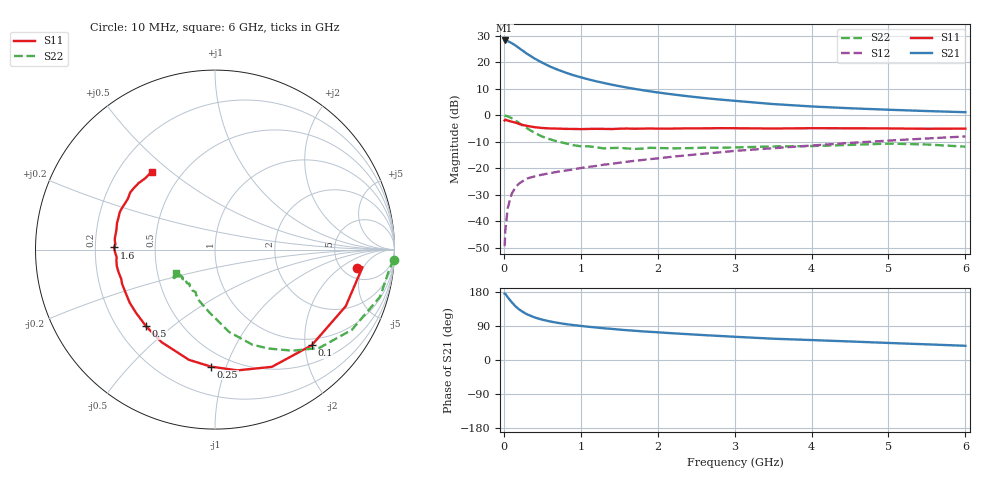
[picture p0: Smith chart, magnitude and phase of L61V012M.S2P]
!  INFINEON TECHNOLOGIES Small Signal Semiconductors
! BFR380L3 , Si-NPN RF-Transistor in TSLP-3-1
!  Vce=1 V,  Ic=12.5 mA
! Common Emitter S-Parameters:  07. March 2005
#  GHz  S  MA  R  50
! f  S11  S21  S12  S22
! GHz  Mag  Ang  Mag  Ang  Mag  Ang  Mag  Ang
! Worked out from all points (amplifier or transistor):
!   36 points, 10 MHz to 6 GHz, reference 50 ohm
!   highest |S21| = 28.2 dB at 10 MHz (marker M1)
!   |S21| within 3 dB of that: start of sweep to 204.1 MHz
!   unconditionally stable (mu >= 1): 1.958 GHz to 4.989 GHz
!   at 250 MHz: K = 0.30, MSG = 24.5 dB, |S12| = -24.7 dB
!   at 1.4 GHz: K = 0.92, MSG = 14.9 dB, |S12| = -18.3 dB
!   at 6 GHz: K = 0.98, MSG = 4.6 dB, |S12| = -8.0 dB
!   S11 on the Smith chart (normalised r, x): 10 MHz: 6.80, -3.73; 100 MHz: 0.86, -2.15; 250 MHz: 0.39, -0.89; 500 MHz: 0.32, -0.41; 1.6 GHz: 0.28, +0.01; 6 GHz: 0.34, +0.43
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0.01  0.7976 -7.2  25.7 175.3  0.0034 86.0  0.9993 -3.2
0.02  0.8273 -6.8  25.59 174.4  0.0069 90.8  0.9769 -6.6
0.05  0.7938 -23.4  24.94 165.7  0.0176 80.1  0.9566 -15.9
0.1  0.7579 -44.7  22.99 153.0  0.0325 69.3  0.8838 -30.4
0.15  0.7261 -64.1  20.74 141.9  0.0438 61.5  0.7985 -43.3
0.2  0.6845 -79.4  18.37 133.2  0.0519 56.3  0.7109 -52.4
0.25  0.6524 -92.0  16.31 126.5  0.058 51.5  0.6273 -61.5
0.3  0.6311 -103.3  14.46 120.7  0.064 49.3  0.5696 -68.5
0.4  0.5954 -120.0  11.72 112.3  0.0704 46.2  0.4644 -80.4
0.5  0.5744 -132.0  9.767 106.4  0.076 45.7  0.396 -87.8
0.6  0.5638 -141.3  8.278 101.7  0.081 45.7  0.3521 -95.0
0.7  0.5599 -148.0  7.225 98.1  0.086 46.6  0.3187 -101.7
0.9  0.5518 -159.8  5.707 92.3  0.095 48.4  0.2731 -112.6
1.1  0.5518 -166.8  4.743 87.7  0.1062 50.7  0.26 -119.1
1.4  0.5495 -175.6  3.774 82.2  0.1211 53.0  0.2409 -127.0
1.6  0.5617 178.8  3.325 78.6  0.1328 54.4  0.2367 -134.6
2.2  0.5607 168.0  2.465 70.4  0.1657 57.2  0.2379 -138.9
2.8  0.57 158.7  1.981 63.5  0.1995 58.8  0.2434 -144.9
3.5  0.5617 149.8  1.624 56.2  0.2392 58.3  0.2577 -144.9
4.5  0.5677 143.0  1.354 48.9  0.3008 58.0  0.2757 -145.0
5.5  0.5558 134.4  1.199 41.3  0.3647 55.1  0.2806 -145.8
6  0.5597 129.0  1.141 37.5  0.398 53.1  0.2558 -149.1
